(* Logix 5000 AddOnInstructionDefinition export AKD_Start_MotionTask; software revision 20.04 *)

TYPE AKD_Status :   // All connections to the drive ethernet module are established and data is successfully transferring.
STRUCT
   Profile_In_Progress : BOOL;   // Profile Move In Progress
   Block_In_Execution : BOOL;   // Block In Execution
   On_Target_Position : BOOL;   // On Target Position (1=Current Position Equals Last Target Position)
   General_Fault : BOOL;   // General Fault
   Current_Direction : BOOL;   // Current Motor Direction (0=Reverse, 1=Forward)
   Home_Level : BOOL;   // Level of Home Input
   Reg_Level : BOOL;   // Level of Registration Input
   Enable : BOOL;   // State of Enable Output
   Fault_Input_Fault : BOOL;   // Fault Input Active
   Fwd_Limit : BOOL;   // Forward Input Active
   Rev_Limit : BOOL;   // Reverse Input Active
   Positive_Limit : BOOL;   // Positive Software Limit Exceeded
   Negative_Limit : BOOL;   // Negative Software Limit Exceeded
   FE_Fault : BOOL;   // Following Error Fault
   Block_Fault : BOOL;   // Block Execution Fault
   Load_Complete : BOOL;   // Command Message Successfully Loaded
END_STRUCT
END_TYPE

TYPE AKD_Control :   // Send Explicit Message
STRUCT
   Load_Data_Start_Profile : BOOL;   // Load Command Data / Start Profile Move
   Start_Block : BOOL;   // Execute Command block or block chain
   Incremental : BOOL;   // Incremental Position (0=Absolute, 1=Incremental)
   Direction : BOOL;   // Direction in Velocity Mode (0=Reverse, 1=Forward)
   Smooth_Stop : BOOL;   // Smooth / Controlled Stop w/ Deceleration
   Hard_Stop : BOOL;   // Hard / Immediate Stop
   Reg_Arm : BOOL;   // Arm the Registration Input
   Enable : BOOL;   // Enable Output
END_STRUCT
END_TYPE

TYPE AKD_Axis :   // Axis Data:
STRUCT
   Control : AKD_Control;   // Control bits to send to the drive
   Status : AKD_Status;   // Status bits received from the drive
   Input : AB:ETHERNET_MODULE_SINT_64Bytes:I:0;   // Data from the drive
   Output : AB:ETHERNET_MODULE_SINT_64Bytes:O:0;   // Data to the drive
   ResponseMsgType : SINT;   // Response type contained in latest IO response from drive. Used to check for errors
   CommandTimeout : INT;   // Time to allow for command response from drive. Dependent on scan rate and communicaiton rate
   PositionFeedback : DINT;   // Actual Position Value
   VelocityFeedback : DINT;   // Actual Velocity Value
END_STRUCT
END_TYPE

ADD_ON_INSTRUCTION AKD_Start_MotionTask   (* revision 2.2, ExecuteEnableInFalse *)
// Revision note:
// Added work around for IN Position bit
// Corrceted for race condition of Start_MT" bit
// Changed IP status to be based on Profile In Progress it instead of not on target position.
// Added N.C. contact for No Profile In Progress status in addition to the existing on target position status to unlatch the Start_Block bit of the control word.
VAR_OUTPUT
   DN : BOOL; {visible}   // Sent Command to Drive
   IP : BOOL; {visible}   // Waiting on Move to finish
   PC : BOOL; {visible}   // Process Complete
   ER : BOOL; {visible}   // Block has error
END_VAR
VAR_IN_OUT
   Axis : AKD_Axis; {required}   // Axis Pointer
END_VAR
VAR_INPUT
   MT_NUM : SINT; {required}   // Motion Task Nymber
   Fault : DINT; {access Read Only, visible}   // Block fault number
END_VAR
VAR
   First_Scan_Bit : BOOL; {access None}
   Function : DINT; {access None}
   Function_Step : DINT; {access None}
   Timer_1 : TIMER := (PRE := 500); {access None}
   dummy : BOOL; {access None}
   Timer_2 : TIMER := (PRE := 100); {access None}
   Timer_3 : TIMER := (PRE := 50); {access None}
END_VAR

ROUTINE EnableInFalse   (* ladder *)
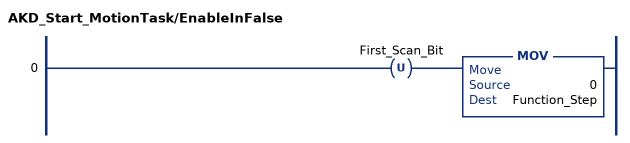
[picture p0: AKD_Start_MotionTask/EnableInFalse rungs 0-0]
   0: OTU(First_Scan_Bit)MOV(0,Function_Step);
END_ROUTINE

ROUTINE Logic   (* ladder *)
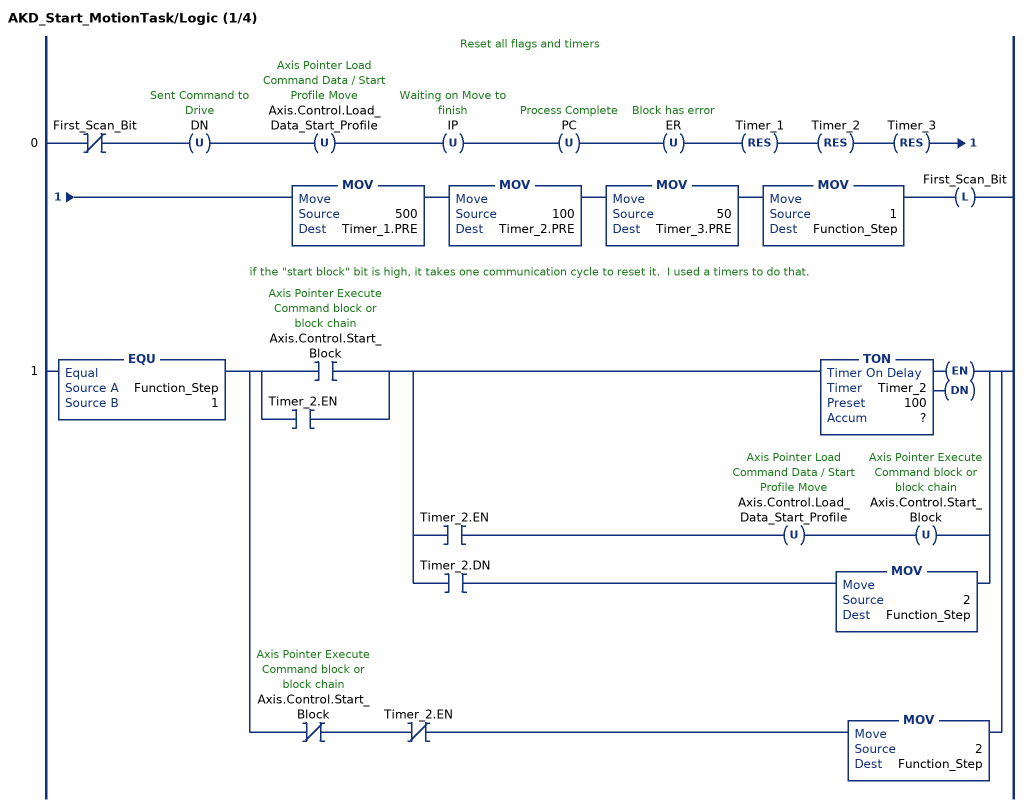
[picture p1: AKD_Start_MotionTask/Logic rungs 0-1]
   // Reset all flags and timers
   0: XIO(First_Scan_Bit)OTU(DN)OTU(Axis.Control.Load_Data_Start_Profile)OTU(IP)OTU(PC)OTU(ER)RES(Timer_1)RES(Timer_2)RES(Timer_3)MOV(500,Timer_1.PRE)MOV(100,Timer_2.PRE)MOV(50,Timer_3.PRE)MOV(1,Function_Step)OTL(First_Scan_Bit);
   // if the "start block" bit is high, it takes one communication cycle to reset it.  I used a timers to do that.
   1: EQU(Function_Step,1)[[XIC(Axis.Control.Start_Block) ,XIC(Timer_2.EN) ] [TON(Timer_2,?,?) ,XIC(Timer_2.EN) OTU(Axis.Control.Load_Data_Start_Profile) OTU(Axis.Control.Start_Block) ,XIC(Timer_2.DN) MOV(2,Function_Step) ] ,XIO(Axis.Control.Start_Block) XIO(Timer_2.EN) MOV(2,Function_Step) ];
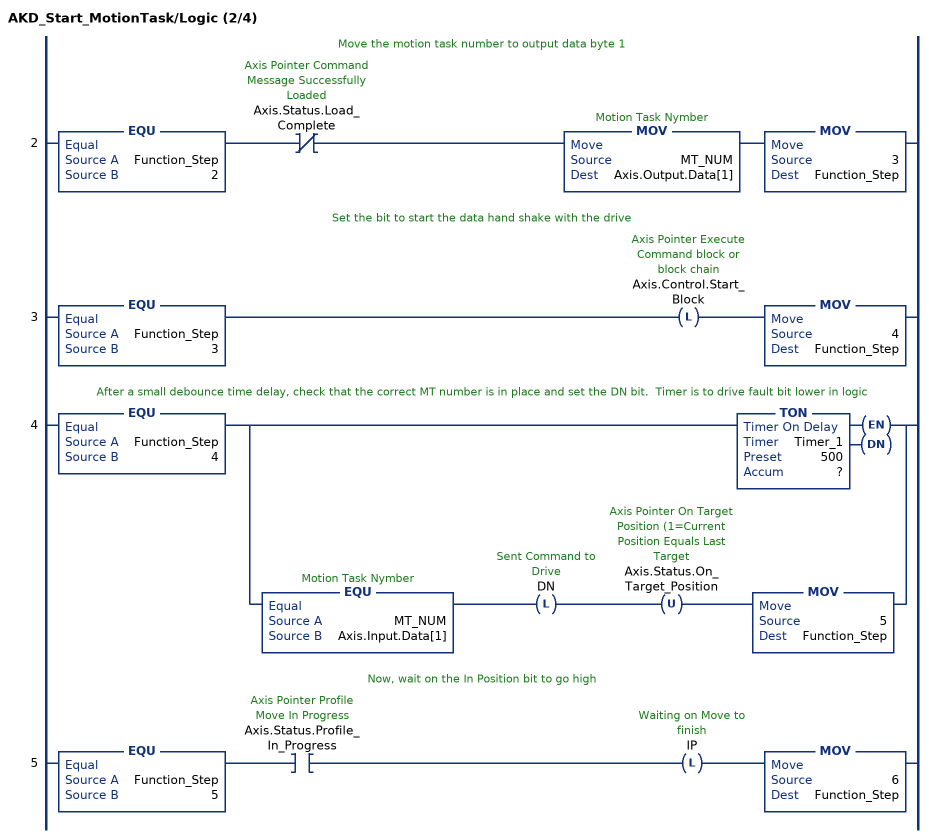
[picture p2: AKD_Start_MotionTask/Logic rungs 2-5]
   // Move the motion task number to output data byte 1
   2: EQU(Function_Step,2)XIO(Axis.Status.Load_Complete)MOV(MT_NUM,Axis.Output.Data[1])MOV(3,Function_Step);
   // Set the bit to start the data hand shake with the drive
   3: EQU(Function_Step,3)OTL(Axis.Control.Start_Block)MOV(4,Function_Step);
   // After a small debounce time delay, check that the correct MT number is in place and set the DN bit.  Timer is to drive fault bit lower in logic
   4: EQU(Function_Step,4)[TON(Timer_1,?,?) ,EQU(MT_NUM,Axis.Input.Data[1]) OTL(DN) OTU(Axis.Status.On_Target_Position) MOV(5,Function_Step) ];
   // Now, wait on the In Position bit to go high
   5: EQU(Function_Step,5)XIC(Axis.Status.Profile_In_Progress)OTL(IP)MOV(6,Function_Step);
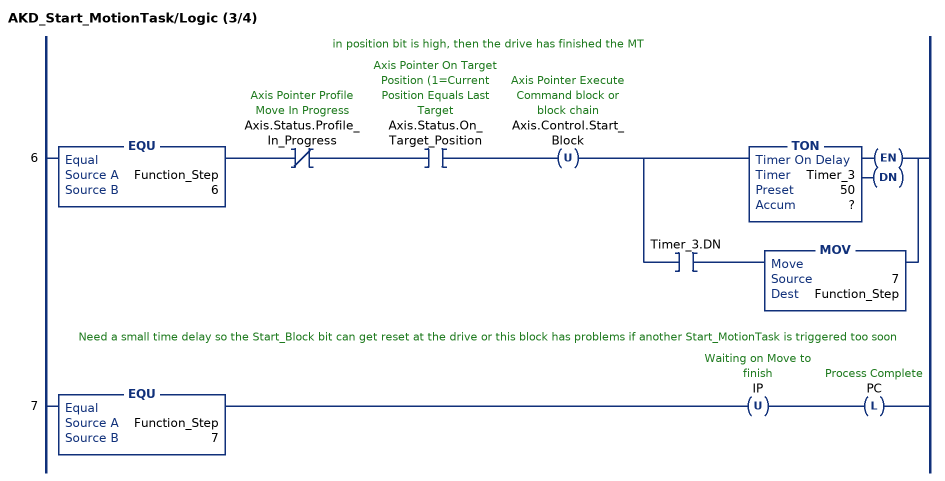
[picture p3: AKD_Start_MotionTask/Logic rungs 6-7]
   // in position bit is high, then the drive has finished the MT
   6: EQU(Function_Step,6)XIO(Axis.Status.Profile_In_Progress)XIC(Axis.Status.On_Target_Position)OTU(Axis.Control.Start_Block)[TON(Timer_3,?,?) ,XIC(Timer_3.DN) MOV(7,Function_Step) ];
   // Need a small time delay so the Start_Block bit can get reset at the drive or this block has problems if another Start_MotionTask is triggered too soon
   7: EQU(Function_Step,7)OTU(IP)OTL(PC);
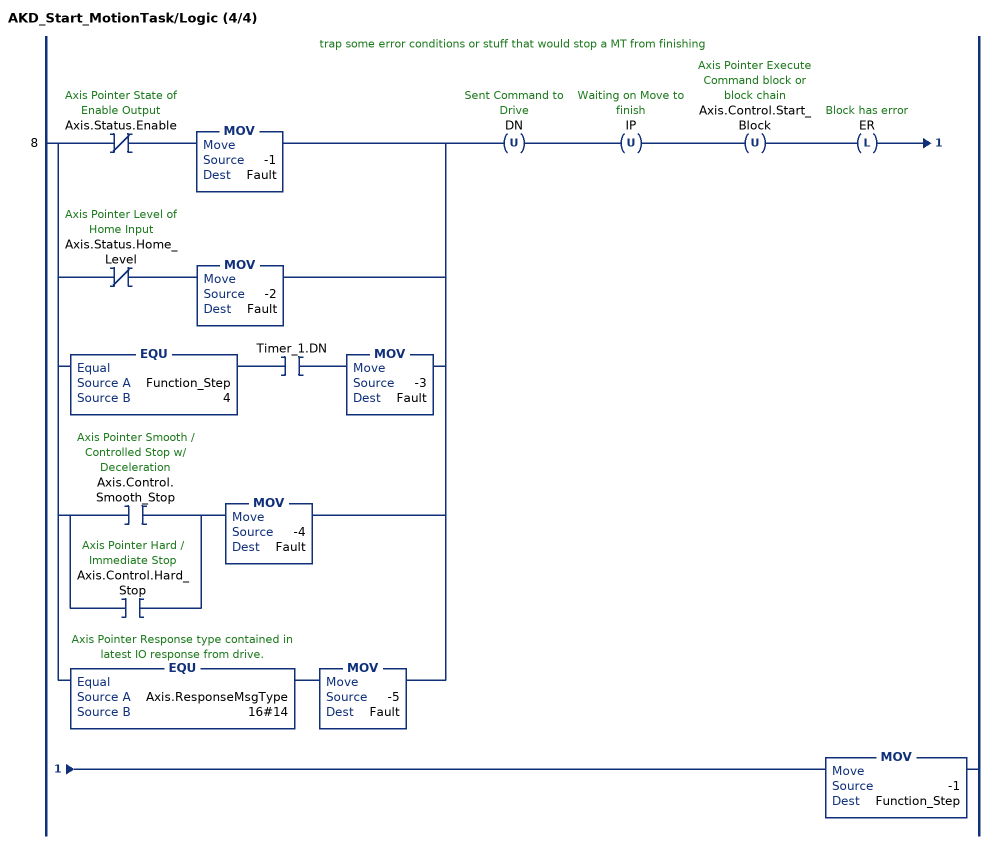
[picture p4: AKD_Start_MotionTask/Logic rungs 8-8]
   // trap some error conditions or stuff that would stop a MT from finishing
   8: [XIO(Axis.Status.Enable) MOV(-1,Fault) ,XIO(Axis.Status.Home_Level) MOV(-2,Fault) ,EQU(Function_Step,4) XIC(Timer_1.DN) MOV(-3,Fault) ,[XIC(Axis.Control.Smooth_Stop) ,XIC(Axis.Control.Hard_Stop) ] MOV(-4,Fault) ,EQU(Axis.ResponseMsgType,16#14) MOV(-5,Fault) ]OTU(DN)OTU(IP)OTU(Axis.Control.Start_Block)OTL(ER)MOV(-1,Function_Step);
END_ROUTINE
END_ADD_ON_INSTRUCTION
